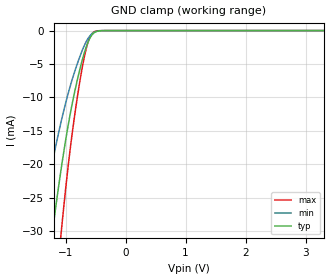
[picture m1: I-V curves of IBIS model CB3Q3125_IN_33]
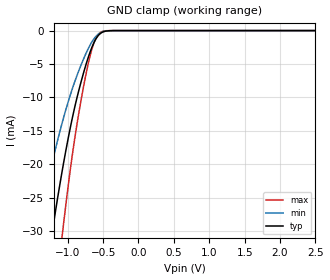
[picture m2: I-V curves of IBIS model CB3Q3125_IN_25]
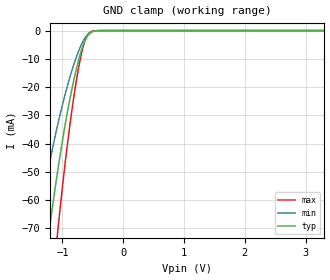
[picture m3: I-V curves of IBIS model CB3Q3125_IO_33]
| TEXAS INSTRUMENTS INCORPORATED
| Standard Linear and Logic Group
| IBIS Model of SN74CB3Q3125
| Quadruple Switch 2.5V/3.3V Low-Voltage, High Bandwitdth FET Bus Switch
| This file contains package information for the following:
|   SSOP 16-pin (DBQ) package as [Component] CB3Q3125_DBQ
|   TVSOP 14-pin (DGV) package as [Component] CB3Q3125_DGV
|   TSSOP 14-pin (PW) package as [Component] CB3Q3125_PW
|   QFN 14-pin (RGY) package as [Component] CB3Q3125_RGY
| This device can be powered at the following Vccs:
|  3.3 volt Vcc
|  2.5 volt Vcc
| This file provides unique models under the [Model Selector] for each Vcc.
| For operation at a specific Vcc, select the appropriate model after each
| [Model Selector] keyword.
[IBIS Ver]   3.2
[Comment char]  |_char
[File Name]   sn74cb3q3125.ibs
[File Rev]   1.2 | b_die
[Date]   February 17, 2004
[Source]   Data created from TI-SPICE simulations at TI-SLL.
[Notes]   The following is an IBIS list for the CB3Q3125.
   Please contact sllibis@ti.com with questions and
   comments concerning SLL IBIS models.
   - FILE REV HISTORY
   - 1.2 Added RGY package on 02/17/04
   - Power-clamp data has been deleted since there is no
   power-clamp diode in the device.
[Disclaimer] Property of Texas Instruments Incorporated.  Unauthorized
   reproduction and/or distribution is strictly prohibited.
   This product is protected under copyright law.
   Created  2003, (C) Copyright  2003, Texas Instruments
   Incorporated, All Rights Reserved
   UNLESS THERE IS A SIGNED, WRITTEN AGREEMENT TO THE
   CONTRARY, TEXAS INSTRUMENTS (TI) IS PROVIDING THE IBIS
   MODELS  AND WITHOUT ANY WARRANTY, EXPRESSED OR
   IMPLIED.  TI assumes no liability for:
   1) the accuracy of the IBIS models provided to your
   company;
   2) the proper functioning of these IBIS Models in your
   design or for any resulting applications; or
   3) infringement of patents, copyrights or intellectual
   property rights resulting from your use of these IBIS
   models.
   TI provides IBIS Models as a service to our customers.
   You and your company shall not distribute, sell or give
   these models to anyone else without prior written
   permission from TI.
   TI reserves the right to make changes to our products or
   to discontinue any semiconductor product or service
   without notice, and advises our customers to obtain the
   latest version of relevant information to verify, before
   placing orders, that the information being relied on is
   current.
   Please be aware that your receipt and use of the IBIS
   information provided shall serve as acceptance of these
   terms and conditions.  If you do not accept these terms,
   you should return or destroy the IBIS models and any
   other accompanying information immediately.
| Component CB3Q3125_DGV 14-pin TVSOP
[Component]   CB3Q3125_DGV
[Manufacturer]   Texas Instruments, Inc.
[Package]
|   typ   min   max
R_pkg   3.500e-02   2.000e-02   4.500e-02
L_pkg   2.499e-09   2.077e-09   2.966e-09
C_pkg   3.610e-13   3.050e-13   4.160e-13
[Pin]   signal_name   model_name   R_pin   L_pin   C_pin
1   1NOE   CB3Q3125_IN   2.700e-02   2.717e-09   3.730e-13
2   1A   CB3Q3125_IO   3.700e-02   2.434e-09   3.980e-13
3   1B   CB3Q3125_IO   3.400e-02   2.200e-09   3.160e-13
4   2NOE   CB3Q3125_IN   2.000e-02   2.077e-09   3.090e-13
5   2A   CB3Q3125_IO   3.000e-02   2.147e-09   3.050e-13
6   2B   CB3Q3125_IO   4.200e-02   2.580e-09   4.080e-13
7   GND   GND   3.900e-02   2.921e-09   3.850e-13
8   3B   CB3Q3125_IO   3.300e-02   2.841e-09   3.800e-13
9   3A   CB3Q3125_IO   4.200e-02   2.611e-09   4.100e-13
10   3NOE   CB3Q3125_IN   3.800e-02   2.331e-09   3.290e-13
11   4B   CB3Q3125_IO   2.600e-02   2.223e-09   3.190e-13
12   4A   CB3Q3125_IO   3.400e-02   2.259e-09   3.130e-13
13   4NOE   CB3Q3125_IN   4.500e-02   2.681e-09   4.160e-13
14   VCC   POWER   4.200e-02   2.966e-09   3.860e-13
| Component CB3Q3125_PW 14-pin TSSOP
[Component]   CB3Q3125_PW
[Manufacturer]   Texas Instruments, Inc.
[Package]
|   typ   min   max
R_pkg   3.200e-02   2.900e-02   3.500e-02
L_pkg   2.378e-09   2.170e-09   2.680e-09
C_pkg   3.140e-13   2.700e-13   3.350e-13
[Pin]   signal_name   model_name   R_pin   L_pin   C_pin
1   1NOE   CB3Q3125_IN   3.300e-02   2.618e-09   3.300e-13
2   1A   CB3Q3125_IO   3.100e-02   2.313e-09   3.170e-13
3   1B   CB3Q3125_IO   3.000e-02   2.310e-09   3.140e-13
4   2NOE   CB3Q3125_IN   3.100e-02   2.173e-09   2.720e-13
5   2A   CB3Q3125_IO   3.000e-02   2.204e-09   3.090e-13
6   2B   CB3Q3125_IO   3.200e-02   2.315e-09   3.170e-13
7   GND   GND   3.500e-02   2.680e-09   3.350e-13
8   3B   CB3Q3125_IO   3.300e-02   2.640e-09   3.330e-13
9   3A   CB3Q3125_IO   3.400e-02   2.347e-09   3.190e-13
10   3NOE   CB3Q3125_IN   2.900e-02   2.277e-09   3.130e-13
11   4B   CB3Q3125_IO   3.100e-02   2.170e-09   2.700e-13
12   4A   CB3Q3125_IO   3.100e-02   2.244e-09   3.110e-13
13   4NOE   CB3Q3125_IN   3.300e-02   2.343e-09   3.210e-13
14   VCC   POWER   3.500e-02   2.657e-09   3.320e-13
| Component CB3Q3125_DBQ 16-pin QSOP
[Component]   CB3Q3125_DBQ
[Manufacturer]   Texas Instruments, Inc.
[Package]
|   typ   min   max
R_pkg   3.800e-02   2.700e-02   5.900e-02
L_pkg   2.353e-09   1.491e-09   4.500e-09
C_pkg   2.100e-13   6.400e-14   5.920e-13
[Pin]   signal_name   model_name   R_pin   L_pin   C_pin
1   NC   NC   5.800e-02   4.450e-09   5.920e-13
2   1NOE   CB3Q3125_IN   4.000e-02   1.930e-09   1.110e-13
3   1A   CB3Q3125_IO   2.800e-02   1.538e-09   7.600e-14
4   1B   CB3Q3125_IO   2.700e-02   1.491e-09   6.400e-14
5   2NOE   CB3Q3125_IN   2.700e-02   1.491e-09   6.400e-14
6   2A   CB3Q3125_IO   2.700e-02   1.506e-09   7.500e-14
7   2B   CB3Q3125_IO   3.300e-02   1.922e-09   1.090e-13
8   GND   GND   5.900e-02   4.500e-09   5.880e-13
9   NC   NC   5.800e-02   3.695e-09   4.140e-13
10   3B   CB3Q3125_IO   3.400e-02   2.685e-09   2.820e-13
11   3A   CB3Q3125_IO   2.900e-02   1.552e-09   7.700e-14
12   3NOE   CB3Q3125_IN   2.800e-02   1.506e-09   6.500e-14
13   4B   CB3Q3125_IO   2.700e-02   1.492e-09   6.400e-14
14   4A   CB3Q3125_IO   2.800e-02   1.534e-09   7.600e-14
15   4NOE   CB3Q3125_IN   4.000e-02   2.703e-09   2.840e-13
16   VCC   POWER   5.600e-02   3.645e-09   4.180e-13
| Component CB3Q3125_RGY 14-pin QFN
[Component]   CB3Q3125_RGY
[Manufacturer]   Texas Instruments, Inc.
[Package]
|   typ   min   max
R_pkg   2.900e-02   2.300e-02   4.100e-02
L_pkg   7.730e-10   6.570e-10   9.980e-10
C_pkg   1.360e-13   1.150e-13   1.560e-13
[Pin]   signal_name   model_name   R_pin   L_pin   C_pin
1   1NOE   CB3Q3125_IN   2.700e-02   8.310e-10   1.300e-13
2   1A   CB3Q3125_IO   2.700e-02   8.660e-10   1.350e-13
3   1B   CB3Q3125_IO   4.100e-02   9.980e-10   1.560e-13
4   2NOE   CB3Q3125_IN   3.100e-02   7.670e-10   1.420e-13
5   2A   CB3Q3125_IO   3.100e-02   7.650e-10   1.420e-13
6   2B   CB3Q3125_IO   3.100e-02   7.830e-10   1.440e-13
7   GND   GND   3.100e-02   7.810e-10   1.370e-13
8   3B   CB3Q3125_IO   2.300e-02   6.570e-10   1.150e-13
9   3A   CB3Q3125_IO   2.300e-02   8.140e-10   1.290e-13
10   3NOE   CB3Q3125_IN   2.800e-02   7.040e-10   1.290e-13
11   4B   CB3Q3125_IO   2.700e-02   6.720e-10   1.360e-13
12   4A   CB3Q3125_IO   2.700e-02   6.960e-10   1.380e-13
13   4NOE   CB3Q3125_IN   2.700e-02   7.250e-10   1.400e-13
14   VCC   POWER   3.000e-02   7.630e-10   1.360e-13
[Series Switch Groups]
| Function Group States
On  1 /   | 1A->1B 1NOE LOW
On  2 /   | 2A->2B 2NOE,LOW
On  3 /   | 3A->3B 3NOE,LOW
On  4 /   | 4A->4B 4NOE,LOW
On  1 2 3 4 /   | Enable All
[Series Pin Mapping]   pin_2   model_name   function_table_group
2   3   CB3Q3125_IO_33_S   1
| 2   3   CB3Q3125_IO_25_S   1
5   6   CB3Q3125_IO_33_S   2
| 5   6   CB3Q3125_IO_25_S   2
8   9   CB3Q3125_IO_33_S   3
| 8   9   CB3Q3125_IO_25_S   3
11   12   CB3Q3125_IO_33_S   4
| 11   12   CB3Q3125_IO_25_S   4
| Model CB3Q3125_IN
[Model Selector]   CB3Q3125_IN
CB3Q3125_IN_33   3.3 volt Vcc
CB3Q3125_IN_25   2.5 volt Vcc
| Model CB3Q3125_IO
[Model Selector]   CB3Q3125_IO
CB3Q3125_IO_33   3.3 volt Vcc
CB3Q3125_IO_25   2.5 volt Vcc
| Model CB3Q3125_IO_S
[Model Selector]   CB3Q3125_IO_S
CB3Q3125_IO_33_S   3.3 volt Vcc
CB3Q3125_IO_25_S   2.5 volt Vcc
[Model]   CB3Q3125_IO_33_S
Model_type  Series_switch
| variable   typ   min   max
C_comp   0   0   0
[Temperature Range]   40   100   -40
| Ambient temperature   25   85   -40
[Voltage range]   3.3   3   3.6
[On]
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[Off]
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[Model]   CB3Q3125_IO_25_S
Model_type  Series_switch
| variable   typ   min   max
C_comp   0   0   0
[Temperature Range]   40   100   -40
| Ambient temperature   25   85   -40
[Voltage range]   2.5   2.3   2.7
[On]
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[Off]
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| Models and submodels in the file (6): CB3Q3125_IN_33 (Input), CB3Q3125_IN_25 (Input), CB3Q3125_IO_33_S (Series_switch), CB3Q3125_IO_33 (Terminator), CB3Q3125_IO_25_S (Series_switch), CB3Q3125_IO_25 (Terminator)
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[Model]   CB3Q3125_IN_33
Model_type  Input
Vinl=0.8
Vinh=2.0
| variable   typ   min   max
C_comp   3.07pF   2.41pF   4.42pF
[Temperature Range]   40   100   -40
| Ambient temperature   25   85   -40
[Voltage range]   3.3   3   3.6
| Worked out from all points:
|   GND clamp passes 1 mA (typ) near -0.59 V on its own axis
[GND Clamp]
| CB3Q3125_IN_33
|   Voltage   I(typ)   I(min)   I(max)
-5.5V     -472.4mA   -358mA     -596.1mA
-1.43V    -45.98mA   -30.17mA   -67.32mA
-1.22V    -30.26mA   -19.79mA   -44.58mA
-1.08V    -21.12mA   -13.88mA   -30.89mA
-1.06V    -19.92mA   -13.1mA    -29.06mA
-975mV    -15.15mA   -10.04mA   -21.76mA
-900mV    -11.44mA   -7.635mA   -16.11mA
-770mV    -6.108mA   -4.099mA   -8.049mA
-645mV    -2.181mA   -1.479mA   -2.339mA
-535mV    -406.2uA   -314.8uA   -251uA
-330mV    -2.055uA   -3.329uA   -188.5nA
3.3V      128.8pA    501.8pA    26.94pA
[Model]   CB3Q3125_IN_25
Model_type  Input
Vinl=0.7
Vinh=1.7
| variable   typ   min   max
C_comp   2.56pF   2.06pF   2.79pF
[Temperature Range]   40   100   -40
| Ambient temperature   25   85   -40
[Voltage range]   2.5   2.3   2.7
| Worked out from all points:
|   GND clamp passes 1 mA (typ) near -0.59 V on its own axis
[GND Clamp]
| CB3Q3125_IN_25
|   Voltage   I(typ)   I(min)   I(max)
-5.5V     -472.4mA   -358mA     -596.1mA
-1.43V    -45.98mA   -30.17mA   -67.32mA
-1.21V    -29.57mA   -19.34mA   -43.56mA
-1.075V   -20.82mA   -13.68mA   -30.43mA
-1.06V    -19.92mA   -13.1mA    -29.06mA
-975mV    -15.15mA   -10.04mA   -21.76mA
-905mV    -11.67mA   -7.786mA   -16.46mA
-780mV    -6.479mA   -4.348mA   -8.607mA
-650mV    -2.304mA   -1.56mA    -2.508mA
-550mV    -541.9uA   -406uA     -369.7uA
-350mV    -3.742uA   -5.538uA   -427.8nA
2.5V      96.07pA    415.1pA    20.34pA
[Model]   CB3Q3125_IO_33
Model_type  Terminator
| variable   typ   min   max
C_comp   4.47pF   3.98pF   5.58pF
| C_tri-state   4.47pF   3.98pF   5.58pF
[Temperature Range]   40   100   -40
| Ambient temperature   25   85   -40
[Voltage range]   3.3   3   3.6
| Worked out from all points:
|   GND clamp passes 1 mA (typ) near -0.55 V on its own axis
[GND Clamp]
| CB3Q3125_IO_33
|   Voltage   I(typ)   I(min)   I(max)
-5.5V     -1.051A    -807.9mA   -1.307A
-1.435V   -107.9mA   -72.65mA   -154.1mA
-1.41V    -103.4mA   -69.56mA   -147.9mA
-1.215V   -70.37mA   -47.15mA   -101.3mA
-1.09V    -51.38mA   -34.48mA   -73.68mA
-1.07V    -48.53mA   -32.59mA   -69.49mA
-925mV    -29.66mA   -20.11mA   -41.47mA
-760mV    -12.65mA   -8.757mA   -16.37mA
-650mV    -4.677mA   -3.352mA   -5.019mA
-555mV    -1.11mA    -859uA     -765.6uA
-330mV    -3.637uA   -5.845uA   -333.9nA
3.3V      197.8pA    862.6pA    19.5pA
